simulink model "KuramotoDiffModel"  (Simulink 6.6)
settings: Solver=ode3  StartTime=0.0  StopTime=Tend  FixedStep=dt  RelTol=1e-8
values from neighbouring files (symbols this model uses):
  k = k+1    (= 1)    [charPathLength.m]    (also in SyncKuramotoDemo.m = 0.2)
  N = length(A)    [charPathLength.m]    (also in DelayDemo.m = 6; PlatoonDemo.m = 40; rlocprint.m = size(R); SelfOrgCopterDemo.m = 7)
  omega = 1    [ConvergenceDemo.m]    (also in PlatoonDemo.m = 0.7; SyncIMPDemo.m = 3; SyncKuramotoDemo.m = [0.4)
  x0 = x0/sum(x0)*N1    [ConsensusDemo.m]    (also in EventtriggeredPendulum.m = [0; 0.18; 0; 0]; LCLCNetworkDemo.m = [x01; zeros((N1-1)*n, 1)]; LCNetworkDemo.m = [1 0 0.5 0 -1 0]; NetwPendulum.m = [0; 0; 0.05; 0])

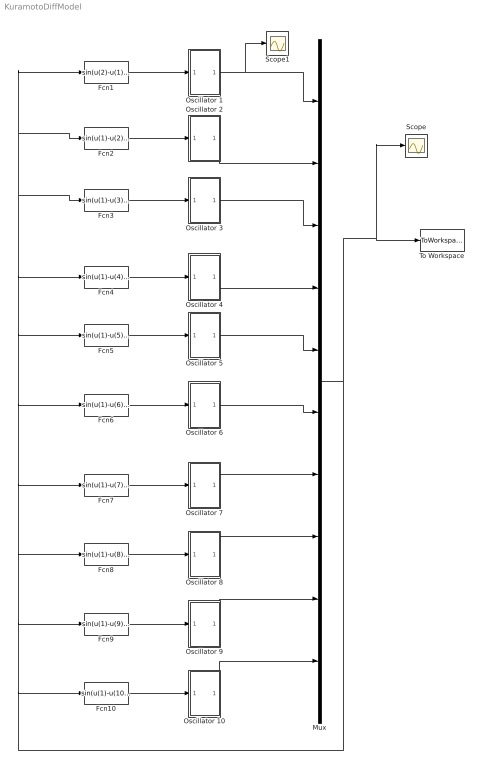
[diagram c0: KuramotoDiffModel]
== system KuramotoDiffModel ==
  Fcn1 : Fcn  Expr=sin(u(2)-u(1))+sin(u(3)-u(1))+sin(u(4)-u(1))+sin(u(5)-u(1))+sin(u(6)-u(1))+sin(u(7)-u(1))+sin(u(8)-u(1))+sin(u(9)-u(1))+sin(u(10)-u(1))
  Fcn10 : Fcn  Expr=sin(u(1)-u(10))+sin(u(2)-u(10))+sin(u(3)-u(10))+sin(u(4)-u(10))+sin(u(5)-u(10))+sin(u(6)-u(10))+sin(u(7)-u(10))+sin(u(8)-u(10))+sin(u(9)-u(10))
  Fcn2 : Fcn  Expr=sin(u(1)-u(2))+sin(u(3)-u(2))+sin(u(4)-u(2))+sin(u(5)-u(2))+sin(u(6)-u(2))+sin(u(7)-u(2))+sin(u(8)-u(2))+sin(u(9)-u(2))+sin(u(10)-u(2))
  Fcn3 : Fcn  Expr=sin(u(1)-u(3))+sin(u(2)-u(3))+sin(u(4)-u(3))+sin(u(5)-u(3))+sin(u(6)-u(3))+sin(u(7)-u(3))+sin(u(8)-u(3))+sin(u(9)-u(3))+sin(u(10)-u(3))
  Fcn4 : Fcn  Expr=sin(u(1)-u(4))+sin(u(2)-u(4))+sin(u(3)-u(4))+sin(u(5)-u(4))+sin(u(6)-u(4))+sin(u(7)-u(4))+sin(u(8)-u(4))+sin(u(9)-u(4))+sin(u(10)-u(4))
  Fcn5 : Fcn  Expr=sin(u(1)-u(5))+sin(u(2)-u(5))+sin(u(3)-u(5))+sin(u(4)-u(5))+sin(u(6)-u(5))+sin(u(7)-u(5))+sin(u(8)-u(5))+sin(u(9)-u(5))+sin(u(10)-u(5))
  Fcn6 : Fcn  Expr=sin(u(1)-u(6))+sin(u(2)-u(6))+sin(u(3)-u(6))+sin(u(4)-u(6))+sin(u(5)-u(6))+sin(u(7)-u(6))+sin(u(8)-u(6))+sin(u(9)-u(6))+sin(u(10)-u(6))
  Fcn7 : Fcn  Expr=sin(u(1)-u(7))+sin(u(2)-u(7))+sin(u(3)-u(7))+sin(u(4)-u(7))+sin(u(5)-u(7))+sin(u(6)-u(7))+sin(u(8)-u(7))+sin(u(9)-u(7))+sin(u(10)-u(7))
  Fcn8 : Fcn  Expr=sin(u(1)-u(8))+sin(u(2)-u(8))+sin(u(3)-u(8))+sin(u(4)-u(8))+sin(u(5)-u(8))+sin(u(6)-u(8))+sin(u(7)-u(8))+sin(u(9)-u(8))+sin(u(10)-u(8))
  Fcn9 : Fcn  Expr=sin(u(1)-u(9))+sin(u(2)-u(9))+sin(u(3)-u(9))+sin(u(4)-u(9))+sin(u(5)-u(9))+sin(u(6)-u(9))+sin(u(7)-u(9))+sin(u(8)-u(9))+sin(u(10)-u(9))
  Mux : Mux  Inputs=10
  Oscillator 1 : Subsystem
  Oscillator 10 : Subsystem
  Oscillator 2 : Subsystem
  Oscillator 3 : Subsystem
  Oscillator 4 : Subsystem
  Oscillator 5 : Subsystem
  Oscillator 6 : Subsystem
  Oscillator 7 : Subsystem
  Oscillator 8 : Subsystem
  Oscillator 9 : Subsystem
  Scope : Scope
  Scope1 : Scope
  To Workspace : ToWorkspace  VariableName=Theta  SampleTime=-1  SaveFormat=Array
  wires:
  Oscillator 1/1(Out1) -> Mux/1, Scope1/1
  Oscillator 2/1(Out1) -> Mux/2
  Oscillator 3/1(Out1) -> Mux/3
  Oscillator 4/1(Out1) -> Mux/4
  Oscillator 5/1(Out1) -> Mux/5
  Oscillator 6/1(Out1) -> Mux/6
  Mux/1 -> To Workspace/1, Scope/1, Fcn1/1, Fcn2/1, Fcn3/1, Fcn4/1, Fcn5/1, Fcn6/1, Fcn7/1, Fcn8/1, Fcn9/1, Fcn10/1
  Fcn1/1 -> Oscillator 1/1(In1)
  Fcn2/1 -> Oscillator 2/1(In1)
  Fcn3/1 -> Oscillator 3/1(In1)
  Fcn4/1 -> Oscillator 4/1(In1)
  Fcn5/1 -> Oscillator 5/1(In1)
  Fcn6/1 -> Oscillator 6/1(In1)
  Oscillator 7/1(Out1) -> Mux/7
  Oscillator 8/1(Out1) -> Mux/8
  Oscillator 9/1(Out1) -> Mux/9
  Oscillator 10/1(Out1) -> Mux/10
  Fcn10/1 -> Oscillator 10/1(In1)
  Fcn9/1 -> Oscillator 9/1(In1)
  Fcn8/1 -> Oscillator 8/1(In1)
  Fcn7/1 -> Oscillator 7/1(In1)

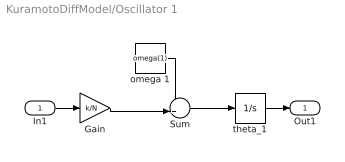
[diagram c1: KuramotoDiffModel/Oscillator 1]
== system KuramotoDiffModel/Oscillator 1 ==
  In1 : Inport
  Gain : Gain  Gain=k/N
  Sum : Sum  Inputs=++|
  omega 1 : Constant  Value=omega(1)
  theta_1 : Integrator  InitialCondition=x0(1)
  Out1 : Outport
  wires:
  omega 1/1 -> Sum/1
  Gain/1 -> Sum/2
  Sum/1 -> theta_1/1
  In1/1 -> Gain/1
  theta_1/1 -> Out1/1

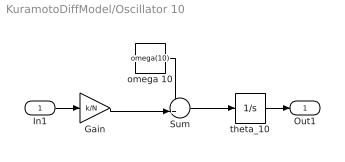
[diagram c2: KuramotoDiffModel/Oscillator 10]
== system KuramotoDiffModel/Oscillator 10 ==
  In1 : Inport
  Gain : Gain  Gain=k/N
  Sum : Sum  Inputs=++|
  omega 10 : Constant  Value=omega(10)
  theta_10 : Integrator  InitialCondition=x0(10)
  Out1 : Outport
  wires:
  omega 10/1 -> Sum/1
  Gain/1 -> Sum/2
  Sum/1 -> theta_10/1
  In1/1 -> Gain/1
  theta_10/1 -> Out1/1

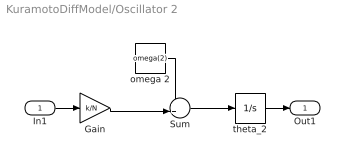
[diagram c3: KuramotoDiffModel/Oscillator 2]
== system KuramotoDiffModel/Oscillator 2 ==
  In1 : Inport
  Gain : Gain  Gain=k/N
  Sum : Sum  Inputs=++|
  omega 2 : Constant  Value=omega(2)
  theta_2 : Integrator  InitialCondition=x0(2)
  Out1 : Outport
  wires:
  omega 2/1 -> Sum/1
  Gain/1 -> Sum/2
  Sum/1 -> theta_2/1
  In1/1 -> Gain/1
  theta_2/1 -> Out1/1

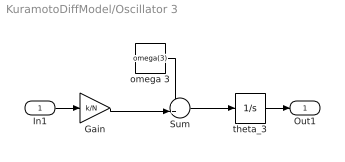
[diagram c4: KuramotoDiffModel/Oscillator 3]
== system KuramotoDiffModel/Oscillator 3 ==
  In1 : Inport
  Gain : Gain  Gain=k/N
  Sum : Sum  Inputs=++|
  omega 3 : Constant  Value=omega(3)
  theta_3 : Integrator  InitialCondition=x0(3)
  Out1 : Outport
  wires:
  omega 3/1 -> Sum/1
  Gain/1 -> Sum/2
  Sum/1 -> theta_3/1
  In1/1 -> Gain/1
  theta_3/1 -> Out1/1

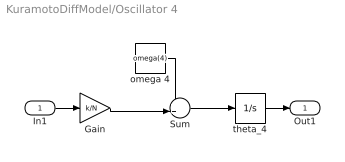
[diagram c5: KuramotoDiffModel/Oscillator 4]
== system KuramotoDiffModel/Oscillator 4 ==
  In1 : Inport
  Gain : Gain  Gain=k/N
  Sum : Sum  Inputs=++|
  omega 4 : Constant  Value=omega(4)
  theta_4 : Integrator  InitialCondition=x0(4)
  Out1 : Outport
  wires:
  omega 4/1 -> Sum/1
  Gain/1 -> Sum/2
  Sum/1 -> theta_4/1
  In1/1 -> Gain/1
  theta_4/1 -> Out1/1

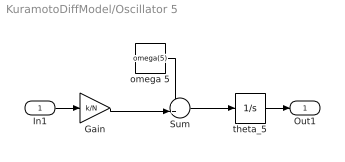
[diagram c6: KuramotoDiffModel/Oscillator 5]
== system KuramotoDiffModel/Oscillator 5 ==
  In1 : Inport
  Gain : Gain  Gain=k/N
  Sum : Sum  Inputs=++|
  omega 5 : Constant  Value=omega(5)
  theta_5 : Integrator  InitialCondition=x0(5)
  Out1 : Outport
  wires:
  omega 5/1 -> Sum/1
  Gain/1 -> Sum/2
  Sum/1 -> theta_5/1
  In1/1 -> Gain/1
  theta_5/1 -> Out1/1

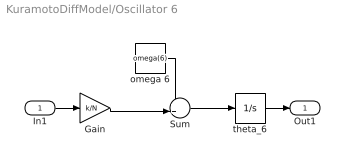
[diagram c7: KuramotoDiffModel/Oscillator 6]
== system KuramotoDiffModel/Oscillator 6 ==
  In1 : Inport
  Gain : Gain  Gain=k/N
  Sum : Sum  Inputs=++|
  omega 6 : Constant  Value=omega(6)
  theta_6 : Integrator  InitialCondition=x0(6)
  Out1 : Outport
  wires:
  omega 6/1 -> Sum/1
  Gain/1 -> Sum/2
  Sum/1 -> theta_6/1
  In1/1 -> Gain/1
  theta_6/1 -> Out1/1

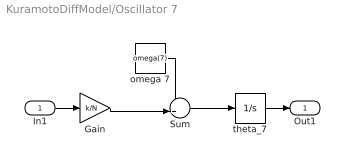
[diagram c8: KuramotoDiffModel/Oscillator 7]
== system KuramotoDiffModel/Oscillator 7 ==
  In1 : Inport
  Gain : Gain  Gain=k/N
  Sum : Sum  Inputs=++|
  omega 7 : Constant  Value=omega(7)
  theta_7 : Integrator  InitialCondition=x0(7)
  Out1 : Outport
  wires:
  omega 7/1 -> Sum/1
  Gain/1 -> Sum/2
  Sum/1 -> theta_7/1
  In1/1 -> Gain/1
  theta_7/1 -> Out1/1

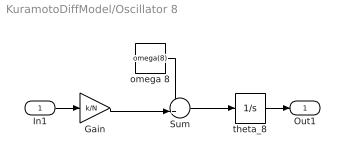
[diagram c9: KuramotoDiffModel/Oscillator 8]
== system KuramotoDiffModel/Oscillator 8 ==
  In1 : Inport
  Gain : Gain  Gain=k/N
  Sum : Sum  Inputs=++|
  omega 8 : Constant  Value=omega(8)
  theta_8 : Integrator  InitialCondition=x0(8)
  Out1 : Outport
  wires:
  omega 8/1 -> Sum/1
  Gain/1 -> Sum/2
  Sum/1 -> theta_8/1
  In1/1 -> Gain/1
  theta_8/1 -> Out1/1

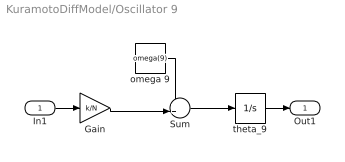
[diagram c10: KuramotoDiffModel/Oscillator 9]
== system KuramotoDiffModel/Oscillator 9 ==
  In1 : Inport
  Gain : Gain  Gain=k/N
  Sum : Sum  Inputs=++|
  omega 9 : Constant  Value=omega(9)
  theta_9 : Integrator  InitialCondition=x0(9)
  Out1 : Outport
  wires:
  omega 9/1 -> Sum/1
  Gain/1 -> Sum/2
  Sum/1 -> theta_9/1
  In1/1 -> Gain/1
  theta_9/1 -> Out1/1
